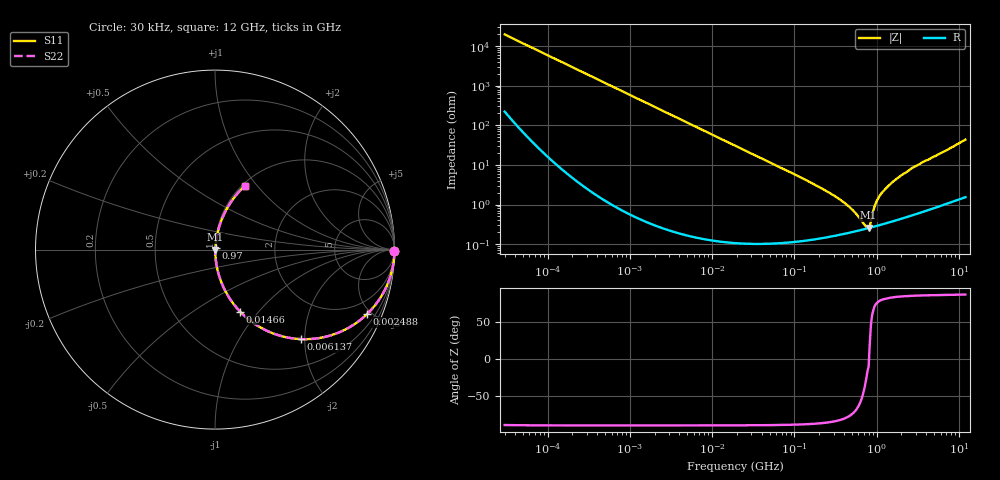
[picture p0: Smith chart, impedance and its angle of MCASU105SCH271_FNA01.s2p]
! MCASU105SCH271_FNA01  S-PARAMETER MODEL  ( General Type )
! Model Generated by TAIYO YUDEN Corporation (http://www.ty-top.com)
! Version 1.0
! TAIYO YUDEN Control No. 130207
! Copyright(c) 2013 TAIYO YUDEN CO.,LTD. All Rights Reserved.
! Product Description (link to TY-COMPAS)
! https://ds.yuden.co.jp/TYCOMPAS/or/detail?pn=MCASU105SCH271JFNA01&u=M
! Products Name : Multilayer Ceramic Capacitors
! Characteristics :
!  Capacitance : 270 pF , Rated Voltage : 50V , TCC : CH / C0H
!  Case Size : 1.0 x 0.5 / 0.039 x 0.02 [mm/inch] , Thickness : 0.5 / 0.02 [mm/inch]
!  (Conditions: Temperature = 25 degC , DC Bias Current/Voltage = 0A / 0V)
! External Node Assignments :
!  1  o---| |---o  2
! GND o---------o GND
! Frequency Range : 30000Hz  -  12GHz  [ 401 STEP ]
# MHz S RI R 50
! Freq[MHz].  S11 Real  S11 Imag  S21 Real  S21 Imag  S12 Real  S12 Imag  S22 Real  S22 Imag
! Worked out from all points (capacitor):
!   401 points, 30 kHz to 12 GHz, reference 50 ohm
!   read as one part in series: C = 270 pF near 32 kHz
!   lowest |Z| = 258 mohm at 799.4 MHz (marker M1)
!   series resonance near 807.4 MHz, so ESL is about 140 pH
!   S11 on the Smith chart (normalised r, x): 30 kHz: open; 2.488 MHz: 1.01, -4.73; 6.137 MHz: 1.00, -1.92; 14.66 MHz: 1.00, -0.80; 970 MHz: 1.01, +0.02; 12 GHz: 1.03, +0.87
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0.03  0.9999 -0.0051  8.37e-05 0.0051  8.37e-05 0.0051  0.9999 -0.0051
0.260295  0.998 -0.0441  0.00201 0.0441  0.00201 0.0441  0.998 -0.0441
0.831097  0.9803 -0.1384  0.0197 0.1384  0.0197 0.1384  0.9803 -0.1384
2.258455  0.8714 -0.3343  0.1286 0.3343  0.1286 0.3343  0.8714 -0.3343
2.487865  0.8481 -0.3584  0.1519 0.3584  0.1519 0.3584  0.8481 -0.3584
4.167822  0.6658 -0.4711  0.3342 0.4711  0.3342 0.4711  0.6658 -0.4711
6.13721  0.4791 -0.4988  0.5209 0.4988  0.5209 0.4988  0.4791 -0.4988
14.65919  0.1394 -0.345  0.8606 0.345  0.8606 0.345  0.1394 -0.345
18.97367  0.0885 -0.2823  0.9115 0.2823  0.9115 0.2823  0.0885 -0.2823
49.92358  0.0146 -0.1156  0.9854 0.1156  0.9854 0.1156  0.0146 -0.1156
164.6252  0.00246 -0.0342  0.9975 0.0342  0.9975 0.0342  0.00246 -0.0342
393.2198  0.00192 -0.0114  0.9981 0.0114  0.9981 0.0114  0.00192 -0.0114
525.6319  0.00209 -0.0065  0.9979 0.0065  0.9979 0.0065  0.00209 -0.0065
725.66  0.00241 -0.00165  0.9976 0.00165  0.9976 0.00165  0.00241 -0.00165
799.3715  0.00254 -0.000444  0.9975 0.000444  0.9975 0.000444  0.00254 -0.000444
852.6267  0.00264 0.00279  0.9974 -0.00279  0.9974 -0.00279  0.00264 0.00279
970.0175  0.00292 0.01  0.9971 -0.01  0.9971 -0.01  0.00292 0.01
1139.739  0.00344 0.0187  0.9966 -0.0187  0.9966 -0.0187  0.00344 0.0187
1428.372  0.00448 0.0306  0.9955 -0.0306  0.9955 -0.0306  0.00448 0.0306
2811.574  0.0129 0.0856  0.9871 -0.0856  0.9871 -0.0856  0.0129 0.0856
6715.658  0.0556 0.2077  0.9444 -0.2077  0.9444 -0.2077  0.0556 0.2077
12000  0.1672 0.356  0.8328 -0.356  0.8328 -0.356  0.1672 0.356
